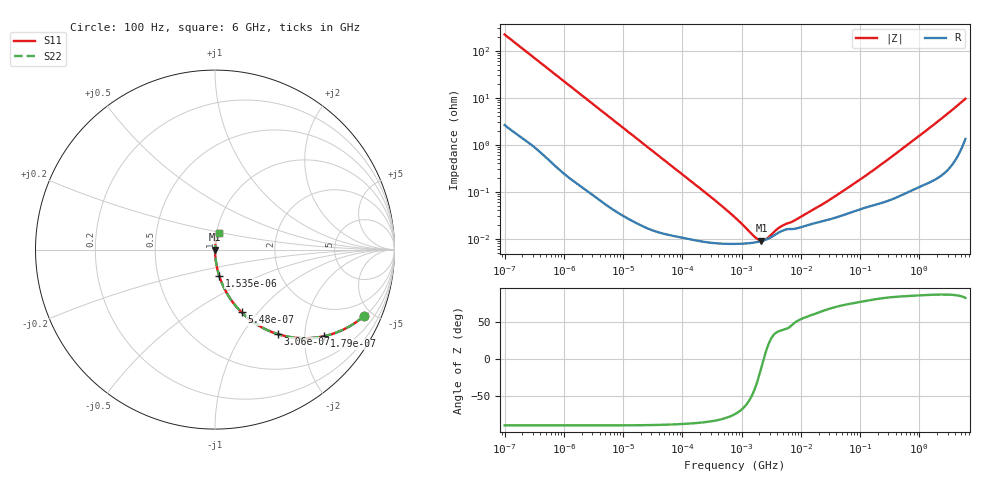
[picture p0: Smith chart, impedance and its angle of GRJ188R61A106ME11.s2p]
!Murata Part Number: GRJ188R61A106ME11
!These Parameters are Measured in Series Mode Connection
!Data Generated on Jun 19, 2026
!  o--ll--o
!Port1  Port2
!  o------o
!Operation Temp=25[degC], DC Bias Voltage=0[V]
!Freq. Start=100[Hz] Stop=6[GHz] 401[Steps]
# Hz S RI R 50
!Freq.(Hz) S11(Real) S11(Imag) S21(Real) S21(Imag) S12(Real) S12(Imag) S22(Real) S22(Imag)
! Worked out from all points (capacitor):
!   401 points, 100 Hz to 6 GHz, reference 50 ohm
!   read as one part in series: C = 7.12 uF near 109 Hz
!   lowest |Z| = 9.06 mohm at 2.169 MHz (marker M1)
!   series resonance near 2.363 MHz, so ESL is about 640 pH
!   S11 on the Smith chart (normalised r, x): 100 Hz: 1.05, -4.46; 179 Hz: 1.03, -2.50; 306 Hz: 1.02, -1.47; 548 Hz: 1.01, -0.82; 1.535 kHz: 1.00, -0.30; 6 GHz: 1.03, +0.19
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100  0.8295 -0.3702  0.1705 0.3702  0.1705 0.3702  0.8295 -0.3702
131  0.742 -0.4317  0.258 0.4317  0.258 0.4317  0.742 -0.4317
179  0.6086 -0.482  0.3914 0.482  0.3914 0.482  0.6086 -0.482
306  0.3519 -0.4713  0.6481 0.4713  0.6481 0.4713  0.3519 -0.4713
548  0.1481 -0.3494  0.8519 0.3494  0.8519 0.3494  0.1481 -0.3494
858  0.0676 -0.2456  0.9324 0.2456  0.9324 0.2456  0.0676 -0.2456
1535  0.023 -0.1445  0.977 0.1445  0.977 0.1445  0.023 -0.1445
2008  0.0139 -0.1117  0.9861 0.1117  0.9861 0.1117  0.0139 -0.1117
6433  0.0017 -0.0356  0.9983 0.0356  0.9983 0.0356  0.0017 -0.0356
40335  0.000169 -0.00575  0.9998 0.00575  0.9998 0.00575  0.000169 -0.00575
316350  8.18e-05 -0.000734  0.9999 0.000734  0.9999 0.000734  8.18e-05 -0.000734
774597  7.74e-05 -0.000273  0.9999 0.000273  0.9999 0.000273  7.74e-05 -0.000273
1658239  8.29e-05 -7.19e-05  0.9999 7.19e-05  0.9999 7.19e-05  8.29e-05 -7.19e-05
2169299  8.9e-05 -1.68e-05  0.9999 1.68e-05  0.9999 1.68e-05  8.9e-05 -1.68e-05
2713602  9.8e-05 2.69e-05  0.9999 -2.69e-05  0.9999 -2.69e-05  9.8e-05 2.69e-05
4643984  0.000143 0.000113  0.9999 -0.000113  0.9999 -0.000113  0.000143 0.000113
7599586  0.000161 0.000176  0.9998 -0.000176  0.9998 -0.000176  0.000161 0.000176
1.555665e7  0.000207 0.000347  0.9998 -0.000347  0.9998 -0.000347  0.000207 0.000347
6.233367e7  0.000345 0.00116  0.9997 -0.00116  0.9997 -0.00116  0.000345 0.00116
3.124326e8  0.00068 0.00507  0.9993 -0.00507  0.9993 -0.00507  0.00068 0.00507
1.873145e9  0.00263 0.0283  0.9974 -0.0283  0.9974 -0.0283  0.00263 0.0283
6e9  0.0216 0.0912  0.9784 -0.0912  0.9784 -0.0912  0.0216 0.0912
